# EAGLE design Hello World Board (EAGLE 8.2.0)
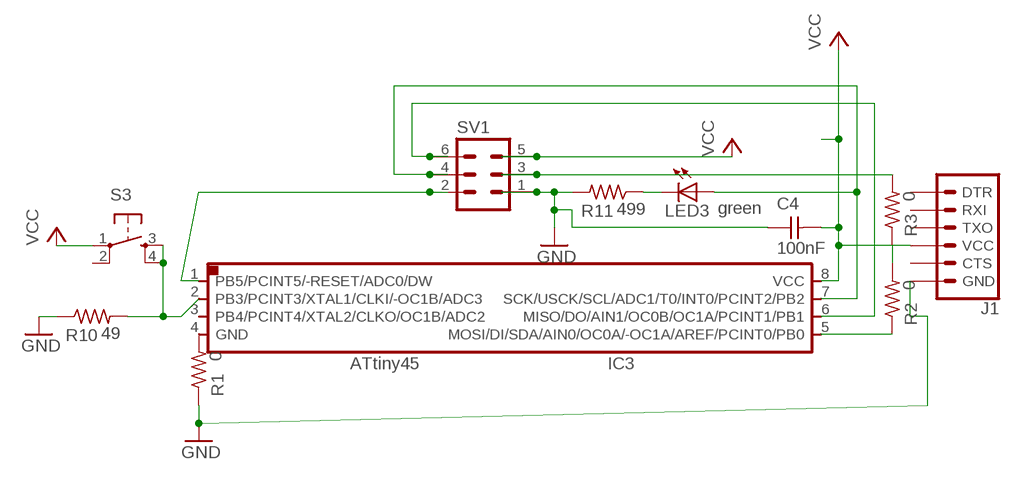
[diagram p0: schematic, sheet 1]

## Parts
C4  100nF  UNPOLARIZED_CAPACITOR1206  [1206]
IC3  ATTINY*5  ATTINY45SI  [SOIC8]
J1  6_PIN_SERIAL_TARGETLONGPADS  [1X06_LONGPADS]
LED3  green  LEDSMT1206  [1206]
R1  0  RESISTOR1206  [1206]
R2  0  RESISTOR1206  [1206]
R3  0  RESISTOR1206  [1206]
R10  49  RESISTOR1206  [1206]
R11  499  RESISTOR1206  [1206]
S3  6MM_SWITCH6MM_SWITCH  [6MM_SWITCH]
SV1  MA03-2  [MA03-2]

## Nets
B2: IC3.2(PB3/PCINT3/XTAL1/CLKI/-OC1B/ADC3) R10.2 S3.3(S) S3.4(S1)
GND: C4.1 J1.6(GND) R1.1 R10.1 R11.2 SV1.1
MISO1: IC3.6(MISO/DO/AIN1/OC0B/OC1A/PCINT1/PB1) SV1.6
MOSI1: R3.2 SV1.3
N$1: IC3.4(GND) R1.2
N$2: IC3.5(MOSI/DI/SDA/AIN0/OC0A/-OC1A/AREF/PCINT0/PB0) R2.1
N$3: R2.2 R3.1
N$5: LED3.C R11.1
RESET1: IC3.1(PB5/PCINT5/-RESET/ADC0/DW) SV1.2
SCK1: IC3.7(SCK/USCK/SCL/ADC1/T0/INT0/PCINT2/PB2) LED3.A SV1.4
VCC: C4.2 IC3.8(VCC) J1.4(VCC) S3.1(P) SV1.5
Unconnected: IC3.3(PB4/PCINT4/XTAL2/CLKO/OC1B/ADC2) J1.1(DTR) J1.2(RXI) J1.3(TXO) J1.5(CTS) S3.2(P1)

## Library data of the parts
C4 = 01_FAB_Hello:UNPOLARIZED_CAPACITOR: unpolarized_capacitor
IC3 = 01_fab:ATTINY45
J1 = SparkFun-Connectors:6_PIN_SERIAL_TARGET: 6-pin header connection for use with the "FTDI BASIC" pinout - TARGET SIDE. Also known as "Arduino Serial Program Header". It is used to mate with our FTDI Basic serial programmers using the Arduino IDE. Note, this device has "TARGET" in the name. It is intended to be used on a design that contains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
LED3 = led:LED: LED
R1-R3 R10 R11 = 01_FAB_Hello:RESISTOR
S3 = 01_fab:6MM_SWITCH: OMRON SWITCH
SV1 = con-lstb:MA03-2: PIN HEADER; OC_FARNELL: unknown; OC_NEWARK: unknown

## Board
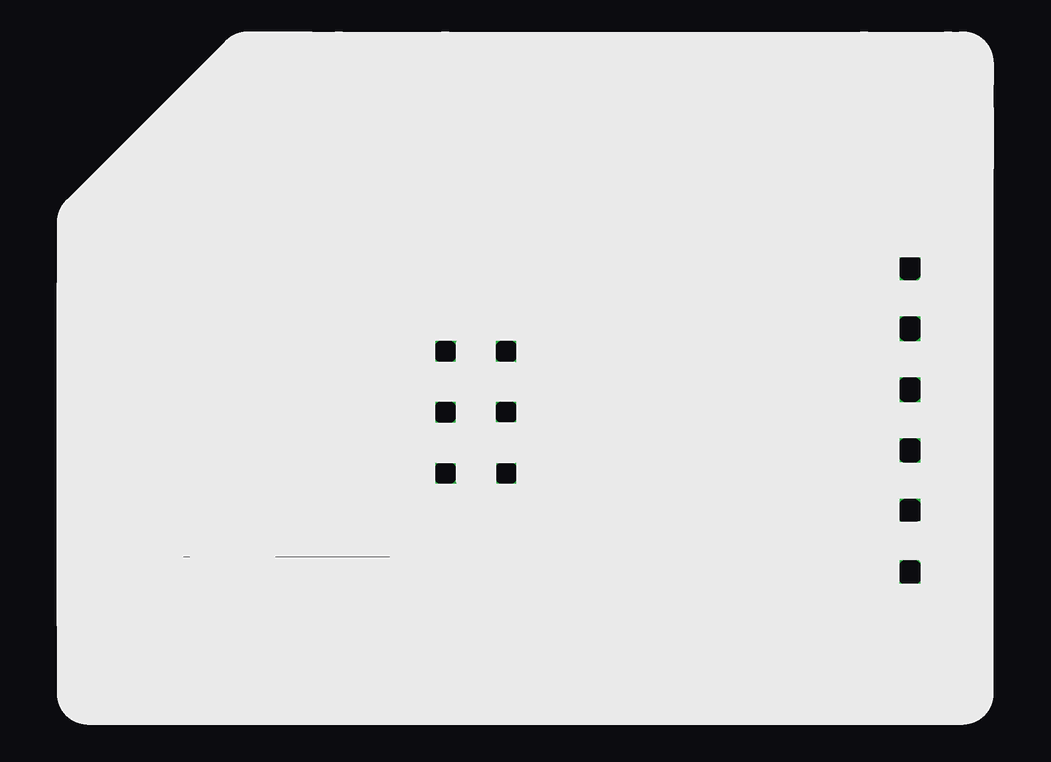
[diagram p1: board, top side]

No outline drawn. Coordinates in mm, seen from the top.
Copper layers (1*16): Top 0.035mm / dielectric 1.5mm / Bottom 0.035mm
Design rules "default *": minimum track width 10mil, minimum drill 24mil, track to track 16mil, track to pad 16mil, pad to pad 16mil, via to via 16mil, smd to smd 8mil, copper to edge 0mil, drill to drill 8mil, minimum pad ring 10mil, minimum via ring 8mil, stop-mask expansion 4mil, vias tented up to drill 0mil, thermal gap 10mil

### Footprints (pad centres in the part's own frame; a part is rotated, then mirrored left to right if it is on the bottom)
1206 = smd 1.6 x 1.803: 1 -1.422,0; 2 1.422,0
SOIC8 = smd 0.5 x 2.2: 1 -1.905,-3.154; 2 -0.645,-3.154; 3 0.625,-3.154; 4 1.895,-3.154; 5 1.905,3.154; 6 0.635,3.154; 7 -0.635,3.154; 8 -1.905,3.154
1X06_LONGPADS = drill 1.118 pad 1.88 long: 1 0,0; 2 2.54,0; 3 5.08,0; 4 7.62,0; 5 10.16,0; 6 12.7,0
1206' = smd 1.6 x 1.803: A -1.422,0; C 1.422,0
6MM_SWITCH = smd 2.286 x 1.524: 1 -3.302,2.286; 2 3.302,2.286; 3 -3.302,-2.286; 4 3.302,-2.286
MA03-2 = drill 1.016: 1 -2.54,-1.27 | drill 1.016 octagon: 2 -2.54,1.27; 3 0,-1.27; 4 0,1.27; 5 2.54,-1.27; 6 2.54,1.27

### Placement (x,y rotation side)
C4  11.43,24.77 180 top
IC3  6.67,12.38 0 top
J1  36.2,19.05 270 top
LED3  green  [1206']  25.08,24.77 180 top
R1  16.83,8.26 180 top
R2  13.02,17.14 90 top
R3  19.37,18.41 0 top
R10  26.99,5.4 180 top
R11  18.23,24.77 180 top
S3  27.94,11.43 270 top
SV1  18.1,13.02 90 top

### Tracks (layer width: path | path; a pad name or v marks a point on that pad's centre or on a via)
B2  (1 unrouted)
  Top 0.406: 25.72,14.92 25.72,15.11 S3.3 25.53,14.61 25.4,14.61 | 25.46,8 25.18,7.8 25.18,13.75 25.72,14.29 25.72,13.97 | 25.46,8 S3.4 25.46,7.94 21.91,7.94 21.91,4.76 15.52,4.72 6.69,4.72 6.39,4.7 6.36,4.72 6.31,4.72 6.27,4.76 5.4,4.76 3.81,6.35 3.81,11.43 6.03,11.43 6.02,11.42 IC3.2 | R10.2 25.57,7.89 25.46,8
GND
  Top 0.406: SV1.1 19.05,10.48 | C4.1 R11.2 16.81,22.91 arc45 16.83,22.86 20.21,22.86 arc-45 20.39,22.79 23.81,19.37 23.81,19.05 | 23.81,19.05 23.81,15.03 arc-45 23.74,14.85 SV1.1 | 23.81,19.05 25.4,19.05 28.34,16.11 arc-45 28.41,15.94 R10.1 31.64,5.4 arc45 31.82,5.47 33.02,6.67 35.77,6.67 arc-45 35.95,6.59 J1.6 | R1.1 19.68,8.26 19.68,10.16 SV1.1
MISO1
  Top 0.406: IC3.6 7.3,17.46 7.62,17.78 9.53,17.78 10.79,17.14 15.56,17.14 SV1.6
MOSI1
  Top 0.406: R3.2 20.95,17.78 21.91,16.83 21.91,15.24 20.64,13.97 20.32,13.97 SV1.3
N$1
  Top 0.406: IC3.4 14.43,9.23 R1.2
N$2
  Top 0.406: IC3.5 12.46,15.54 arc-45 12.64,15.46 R2.1
N$3
  Top 0.406: R2.2 17.69,18.57 arc-45 17.87,18.49 R3.1
N$5
  Top 0.406: R11.1 LED3.C
RESET1
  Top 0.406: 4.76,8.89 IC3.1 4.84,8.83 4.84,7.02 6.65,5.54 15.26,5.54 16.83,6.15 SV1.2
SCK1
  Top 0.406: IC3.7 6.03,13.02 8.26,13.02 8.89,13.65 13.65,13.65 14.29,13.02 SV1.4
  Top 0.508: LED3.A 26.5,22.71 27.94,21.27 38.42,21.27 39.05,20.64 39.05,4.76 38.1,3.81 6.2,3.81 6.12,3.8 | 6.12,3.8 | 6.12,3.8 4.14,3.8 4.13,3.81 1.27,6.67 1.27,13.02 6.03,13.02
VCC
  Top 0.406: 4.76,15.88 IC3.8 | IC3.8 4.78,15.24 4.76,15.24 | C4.2 4.76,24.77 IC3.8 | 19.68,15.88 19.59,15.97 19.59,16.41 19.37,16.19 SV1.5 19.37,20.95 11.43,20.95 10.01,22.38 C4.2 | C4.2 10.01,25.25 12.06,27.3 24.13,27.3 25.08,26.35 25.08,23.62 25.13,21.98 25.32,21.67 30.48,16.51 30.48,14.99 S3.1 31.62,14.73 34.29,12.06 35.56,12.06 J1.4

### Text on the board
Top: Hello World - FabLab Rwanda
